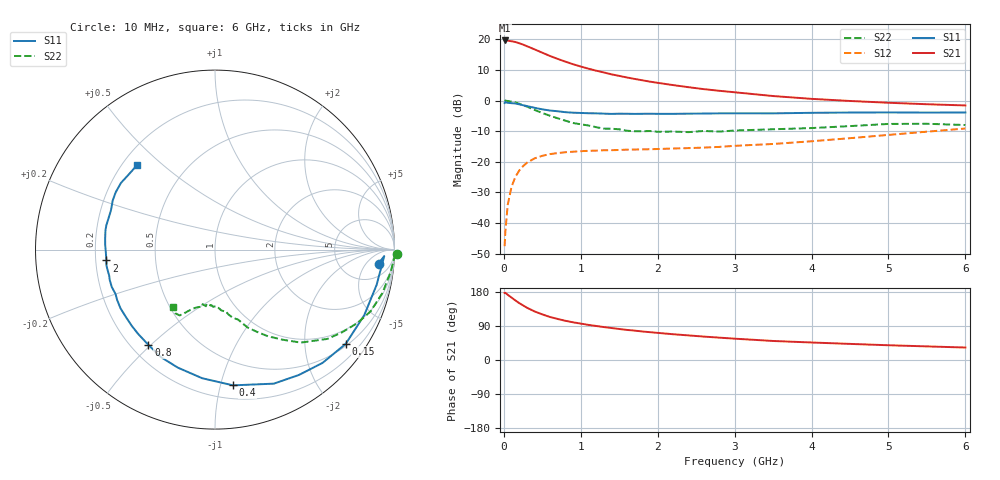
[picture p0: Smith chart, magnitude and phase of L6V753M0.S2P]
!  INFINEON TECHNOLOGIES Small Signal Semiconductors
! BFR380L3 , Si-NPN RF-Transistor in TSLP-3-1
!  Vce=0.75 V,  Ic=3 mA
! Common Emitter S-Parameters:  07. March 2005
#  GHz  S  MA  R  50
! f  S11  S21  S12  S22
! GHz  Mag  Ang  Mag  Ang  Mag  Ang  Mag  Ang
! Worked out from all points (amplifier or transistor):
!   36 points, 10 MHz to 6 GHz, reference 50 ohm
!   highest |S21| = 19.6 dB at 10 MHz (marker M1)
!   |S21| within 3 dB of that: start of sweep to 408 MHz
!   unconditionally stable (mu >= 1): 2.497 GHz to 4.916 GHz
!   at 250 MHz: K = 0.12, MSG = 19.8 dB, |S12| = -21.4 dB
!   at 1.4 GHz: K = 0.67, MSG = 12.4 dB, |S12| = -16.2 dB
!   at 6 GHz: K = 0.97, MSG = 3.8 dB, |S12| = -9.1 dB
!   S11 on the Smith chart (normalised r, x): 10 MHz: 12, -11; 150 MHz: 0.55, -3.00; 400 MHz: 0.30, -1.10; 800 MHz: 0.27, -0.49; 2 GHz: 0.24, -0.05; 6 GHz: 0.26, +0.41
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0.01  0.9146 -4.9  9.605 176.9  0.0042 86.4  1.012 -1.5
0.02  0.9436 -2.2  9.547 177.3  0.0073 87.0  0.9977 -3.1
0.05  0.9217 -12.3  9.542 172.2  0.0197 83.7  0.9866 -7.4
0.1  0.9083 -23.7  9.319 164.7  0.0392 76.6  0.9634 -14.6
0.15  0.8979 -35.8  9.064 157.2  0.0569 70.5  0.9326 -21.7
0.2  0.8703 -46.5  8.651 150.1  0.0721 66.0  0.8917 -27.4
0.25  0.8405 -56.2  8.219 144.1  0.0852 60.2  0.8421 -33.4
0.3  0.8156 -66.3  7.742 138.0  0.0967 55.8  0.7994 -38.5
0.4  0.7631 -82.4  6.868 128.1  0.114 48.5  0.7051 -47.3
0.5  0.7202 -95.7  6.061 120.4  0.1254 43.2  0.6278 -53.1
0.6  0.6894 -107.5  5.359 113.5  0.1338 39.3  0.5658 -58.6
0.8  0.6476 -125.0  4.332 103.5  0.1436 34.6  0.4705 -67.3
0.9  0.6353 -132.6  3.928 99.4  0.1464 33.1  0.4311 -70.1
1.1  0.6222 -143.2  3.323 92.6  0.1515 31.6  0.3927 -75.4
1.5  0.6117 -160.1  2.535 81.8  0.1564 31.2  0.3399 -84.2
2  0.6083 -174.3  1.952 71.6  0.1621 34.0  0.3097 -93.7
2.2  0.6083 -178.4  1.794 68.0  0.1652 35.5  0.3125 -94.2
2.8  0.6197 170.1  1.448 59.0  0.1755 41.4  0.3119 -102.8
3.5  0.6194 159.5  1.188 50.2  0.196 47.1  0.3406 -108.3
4.5  0.6388 150.0  0.987 42.5  0.2436 55.1  0.3838 -114.7
5.5  0.6374 139.0  0.873 35.9  0.3111 57.6  0.4186 -121.7
6  0.6403 132.6  0.834 32.9  0.3505 57.1  0.3996 -126.3
